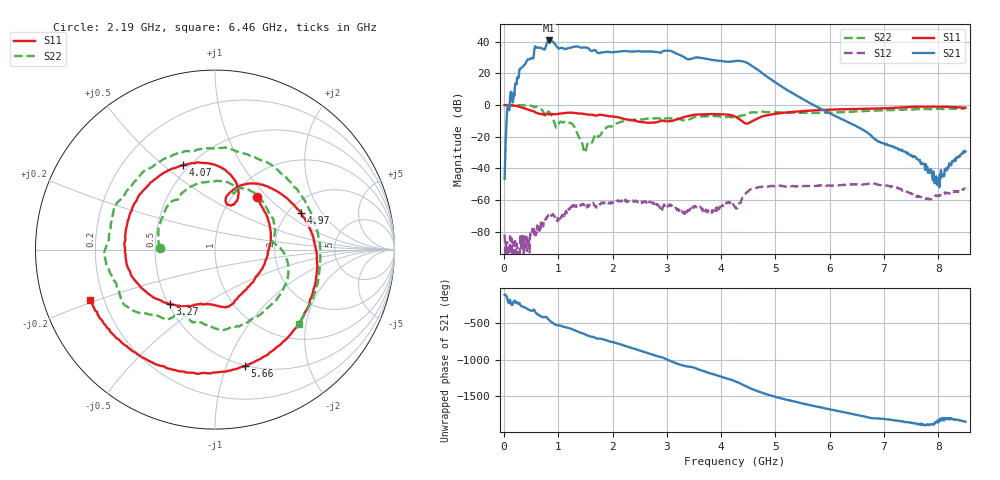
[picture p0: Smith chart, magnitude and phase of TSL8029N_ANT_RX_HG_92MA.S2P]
!Agilent Technologies,E5071C,MY46523237,B.13.01
!Date: Wed Oct 18 11:27:38 2023
!Data & Calibration Information:
!Freq	S11:SOLT2(ON)	S21:SOLT2(ON)	S12:SOLT2(ON)	S22:SOLT2(ON)
!PortZ  Port1:50+j0  Port2:50+j0
!Above PortZ is port z conversion or system Z0 setting when saving the data.
!When reading, reference impedance value at option line is always used.
# Hz S dB R 50
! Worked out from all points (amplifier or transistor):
!   850 points, 10 MHz to 8.5 GHz, reference 50 ohm
!   highest |S21| = 40.8 dB at 830 MHz (marker M1)
!   |S21| within 3 dB of that: 776.1 MHz to 954.6 MHz (178.6 MHz wide, 20.6 % of centre)
!   unconditionally stable (mu >= 1): 16.3 MHz to 28.65 MHz; 73.76 MHz to 101.9 MHz; 121.4 MHz to end of sweep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
!   at 1.42 GHz: K = 8.01, MAG = 37.7 dB, |S12| = -63.3 dB
!   at 4.26 GHz: K = 23.81, MAG = 29.5 dB, |S12| = -64.7 dB
!   at 8.5 GHz: K = 777.65, MAG = -20.2 dB, |S12| = -52.7 dB
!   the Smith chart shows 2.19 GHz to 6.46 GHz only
!   S11 on the Smith chart (normalised r, x): 2.19 GHz: 1.27, +0.87; 3.27 GHz: 0.51, -0.37; 4.07 GHz: 0.46, +0.59; 4.97 GHz: 2.32, +1.30; 5.66 GHz: 0.49, -1.16; 6.46 GHz: 0.15, -0.19
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1e7  -0.00 -2.0  -46.61 -118.4  -81.81 156.6  0.04 -1.9
5.3e8  -3.80 -92.3  29.35 26.4  -80.36 -91.8  -0.73 -111.1
6.1e8  -5.05 -101.2  36.13 -17.9  -76.10 -147.4  -1.19 -129.0
8.3e8  -5.80 -115.3  40.82 -100.8  -70.27 119.8  -4.30 -172.8
9.3e8  -5.76 -125.2  38.84 -157.0  -70.46 85.9  -11.46 156.5
1.25e9  -4.81 -165.7  36.51 135.0  -63.59 52.7  -11.82 133.3
1.43e9  -5.44 169.3  36.26 81.7  -62.92 9.8  -23.12 80.5
1.68e9  -6.72 135.9  34.66 15.1  -64.06 -40.5  -18.54 -128.5
2.19e9  -8.54 51.6  34.17 -83.5  -60.45 -99.9  -10.24 178.7
2.53e9  -10.72 -9.4  33.89 -163.5  -62.00 -141.3  -9.08 127.8
2.84e9  -10.58 -64.3  33.40 122.4  -63.39 166.5  -8.37 82.0
3.02e9  -10.32 -98.1  34.39 76.0  -63.67 156.5  -8.33 57.3
3.27e9  -8.09 -129.6  31.11 5.1  -66.83 131.1  -9.25 14.8
3.68e9  -5.88 165.7  29.51 -78.6  -65.64 103.4  -7.17 -46.1
4.07e9  -5.97 110.6  27.52 -170.3  -62.47 109.1  -7.70 -102.8
4.26e9  -7.31 79.3  27.83 144.1  -64.72 82.0  -7.84 -118.7
4.97e9  -5.69 23.3  14.95 -61.5  -51.32 -19.4  -4.35 155.9
5.66e9  -3.48 -75.5  0.81 174.7  -51.15 -120.3  -5.05 65.3
5.67e9  -3.47 -76.9  0.62 173.5  -51.07 -121.6  -5.05 64.1
6.46e9  -2.49 -157.8  -12.88 51.4  -50.09 129.4  -4.09 -41.7
7.09e9  -1.91 144.7  -25.45 -16.9  -51.16 23.2  -3.15 -114.5
8.5e9  -1.68 -20.9  -29.25 -47.5  -52.72 44.8  -2.12 92.3
